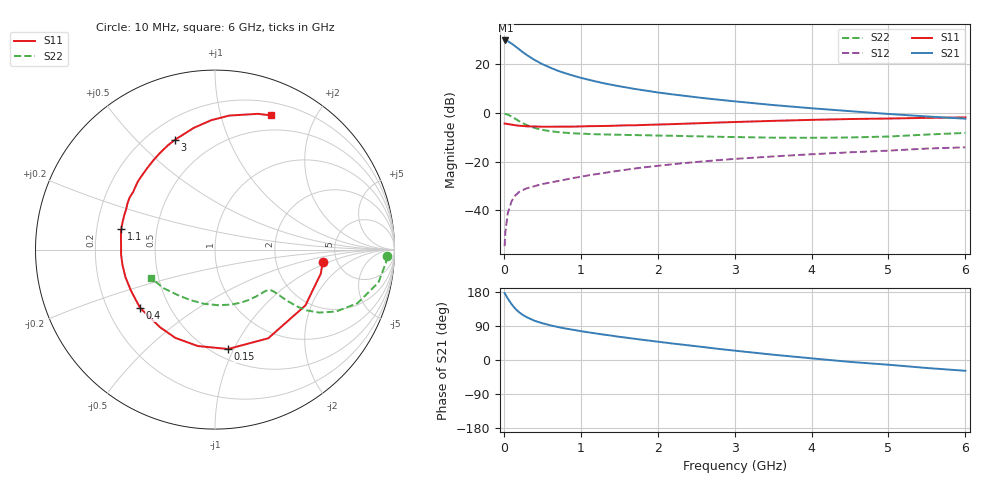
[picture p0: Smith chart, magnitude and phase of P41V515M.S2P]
! SIEMENS Small Signal Semiconductors
! BFP182
! Si NPN RF Bipolar Junction Transistor in SOT143
! VCE = 1.5 V  IC = 15 mA
! Common Emitter S-Parameters:  March  1996
# GHz  S  MA  R  50
!  f  S11  S21  S12  S22
! GHz  MAG  ANG  MAG  ANG  MAG  ANG  MAG  ANG
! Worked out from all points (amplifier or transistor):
!   36 points, 10 MHz to 6 GHz, reference 50 ohm
!   highest |S21| = 29.9 dB at 20 MHz (marker M1)
!   |S21| within 3 dB of that: start of sweep to 173.1 MHz
!   unconditionally stable (mu >= 1): 729.2 MHz to 5.619 GHz
!   at 250 MHz: K = 0.47, MSG = 28.3 dB, |S12| = -31.7 dB
!   at 1.4 GHz: K = 1.23, MAG = 15.1 dB, |S12| = -24.2 dB
!   at 6 GHz: K = 0.97, MSG = 5.9 dB, |S12| = -14.1 dB
!   S11 on the Smith chart (normalised r, x): 10 MHz: 3.86, -0.83; 150 MHz: 0.59, -0.95; 400 MHz: 0.34, -0.31; 1.1 GHz: 0.31, +0.10; 3 GHz: 0.31, +0.66; 6 GHz: 0.33, +1.45
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0.01  0.604 -6.5  31.1 176.6  0.0018 82.0  0.9595 -2.2
0.02  0.6044 -12.8  31.27 173.3  0.0035 83.8  0.9545 -4.5
0.05  0.592 -31.7  30.29 162.5  0.0085 79.2  0.9286 -11.4
0.1  0.5763 -59.0  27.01 147.5  0.0151 65.1  0.8483 -20.6
0.15  0.5586 -82.5  23.65 135.1  0.0201 57.6  0.7577 -27.1
0.2  0.5458 -100.1  20.49 125.8  0.0237 52.8  0.6774 -31.2
0.25  0.5392 -114.2  17.75 118.4  0.026 49.5  0.6134 -33.5
0.3  0.5301 -125.3  15.6 112.7  0.0281 47.9  0.5619 -34.6
0.4  0.5289 -142.1  12.39 103.5  0.0311 46.2  0.4922 -35.4
0.5  0.5212 -153.6  10.16 97.1  0.0343 45.8  0.4498 -35.4
0.6  0.5221 -162.9  8.664 91.7  0.0368 46.4  0.4231 -35.4
0.7  0.5227 -170.7  7.43 87.1  0.0395 47.5  0.4042 -35.5
0.9  0.5239 177.4  5.899 79.7  0.0457 49.0  0.3814 -36.2
1.1  0.535 167.8  4.856 72.9  0.0519 49.9  0.3697 -38.0
1.3  0.5405 159.4  4.099 67.0  0.0581 50.1  0.3615 -40.2
1.5  0.5511 152.4  3.558 61.2  0.0648 50.2  0.3561 -43.0
2.2  0.5899 130.0  2.412 43.3  0.0881 47.2  0.3396 -55.3
3  0.6515 109.9  1.739 24.7  0.1132 41.1  0.3195 -73.6
3.5  0.6884 99.9  1.459 14.0  0.1271 36.9  0.3101 -87.0
4.5  0.7511 83.9  1.091 -5.0  0.1547 28.6  0.313 -116.0
5.5  0.7936 72.4  0.849 -21.1  0.1848 20.4  0.3593 -143.5
6  0.8108 67.2  0.763 -28.5  0.1963 15.2  0.3888 -156.0
